FUNCTION "FC_CONVEYORS" : VOID
TITLE =FC DATA EXCHANGE WITH CONVEYOR SYSTEM
{ S7_language := '9(1) Angielski (Stany Zjednoczone)  11.01.2022  09:45:15' }
VERSION : 0.1


VAR_TEMP
  DoorOK : BOOL ;	//ASU COOLING ZONE DOORS OK (CLOSED)
  RET_VAL_IN : INT ;
  RET_VAL_OUT : INT ;
  T_Pos : BOOL ;
  T_Neg : BOOL ;
  FullProd15_Plus1 : REAL ;
  FullProd15_Minus1 : REAL ;
  FullProd20_Plus1 : REAL ;
  FullProd20_Minus1 : REAL ;
END_VAR
BEGIN
NETWORK
TITLE =*********** START ************
//
//******************** INPUT SIGNALS (FROM CONVEYORS) ***************************
//
NETWORK
TITLE =READ DATA FROM CONVEYORS
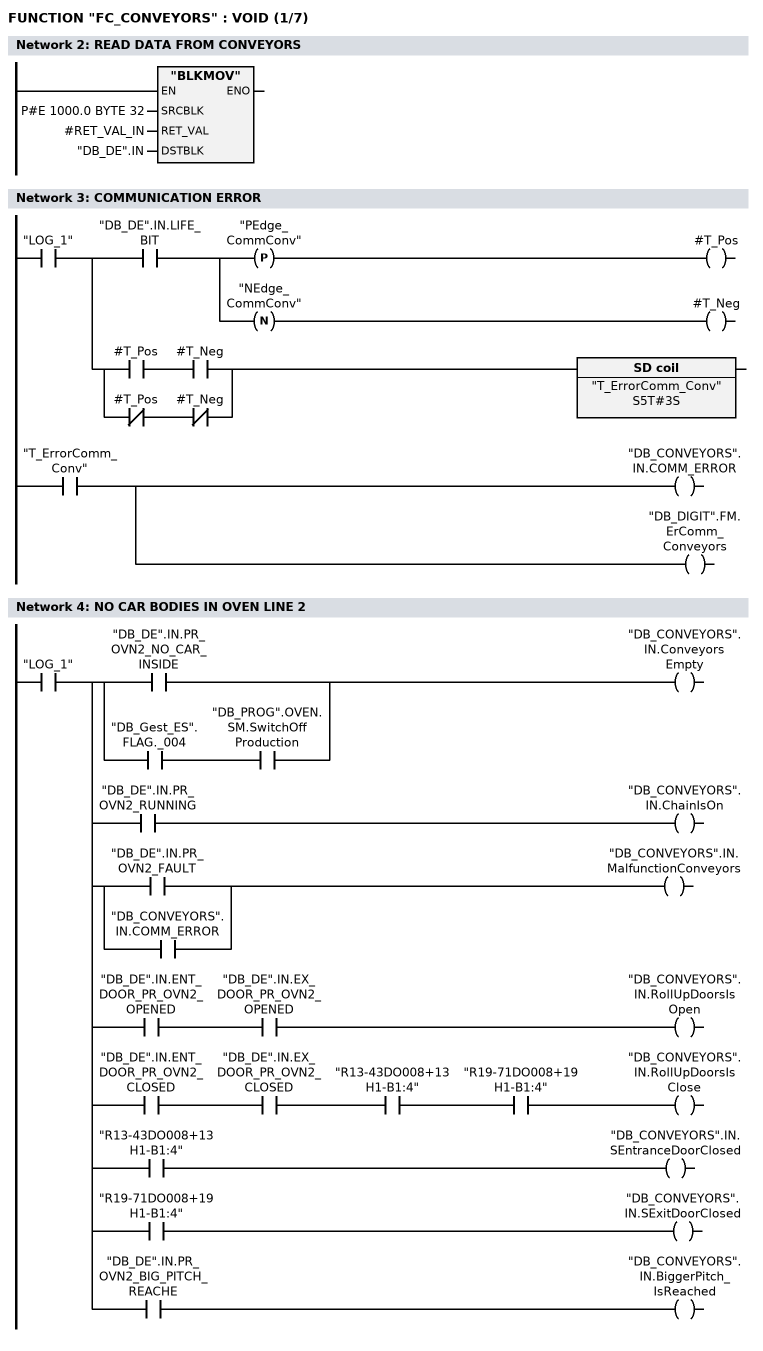
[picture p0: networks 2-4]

      CALL "BLKMOV" (
           SRCBLK                   := P#E 1000.0 BYTE 32,
           RET_VAL                  := #RET_VAL_IN,
           DSTBLK                   := "DB_DE".IN);
      NOP   0;
NETWORK
TITLE =COMMUNICATION ERROR

      U     "LOG_1";
      =     L     24.0;
      U     L     24.0;
      U     "DB_DE".IN.LIFE_BIT;
      =     L     24.1;
      U     L     24.1;
      FP    "PEdge_CommConv";
      =     #T_Pos;
      U     L     24.1;
      FN    "NEdge_CommConv";
      =     #T_Neg;
      U     L     24.0;
      U(    ;
      U     #T_Pos;
      U     #T_Neg;
      O     ;
      UN    #T_Pos;
      UN    #T_Neg;
      )     ;
      L     S5T#3S;
      SE    "T_ErrorComm_Conv";
      NOP   0;
      NOP   0;
      NOP   0;
      U     "T_ErrorComm_Conv";
      =     "DB_CONVEYORS".IN.COMM_ERROR;
      =     "DB_DIGIT".FM.ErComm_Conveyors;
NETWORK
TITLE =NO CAR BODIES IN OVEN LINE 2

      U     "LOG_1";
      =     L     24.0;
      U     L     24.0;
      U(    ;
      O     "DB_DE".IN.PR_OVN2_NO_CAR_INSIDE;
      O     ;
      U     "DB_Gest_ES".FLAG._004;
      U     "DB_PROG".OVEN.SM.SwitchOffProduction;
      )     ;
      =     "DB_CONVEYORS".IN.ConveyorsEmpty;
      U     L     24.0;
      U     "DB_DE".IN.PR_OVN2_RUNNING;
      =     "DB_CONVEYORS".IN.ChainIsOn;
      U     L     24.0;
      U(    ;
      O     "DB_DE".IN.PR_OVN2_FAULT;
      O     "DB_CONVEYORS".IN.COMM_ERROR;
      )     ;
      =     "DB_CONVEYORS".IN.MalfunctionConveyors;
      U     L     24.0;
      U     "DB_DE".IN.ENT_DOOR_PR_OVN2_OPENED;
      U     "DB_DE".IN.EX_DOOR_PR_OVN2_OPENED;
      =     "DB_CONVEYORS".IN.RollUpDoorsIsOpen;
      U     L     24.0;
      U     "DB_DE".IN.ENT_DOOR_PR_OVN2_CLOSED;
      U     "DB_DE".IN.EX_DOOR_PR_OVN2_CLOSED;
      U     "R13-43DO008+13H1-B1:4";
      U     "R19-71DO008+19H1-B1:4";
      =     "DB_CONVEYORS".IN.RollUpDoorsIsClose;
      U     L     24.0;
      U     "R13-43DO008+13H1-B1:4";
      =     "DB_CONVEYORS".IN.SEntranceDoorClosed;
      U     L     24.0;
      U     "R19-71DO008+19H1-B1:4";
      =     "DB_CONVEYORS".IN.SExitDoorClosed;
      U     L     24.0;
      U     "DB_DE".IN.PR_OVN2_BIG_PITCH_REACHE;
      =     "DB_CONVEYORS".IN.BiggerPitch_IsReached;
NETWORK
TITLE =ROLL UP DOOR ENTRANCE IS MOVED FREE
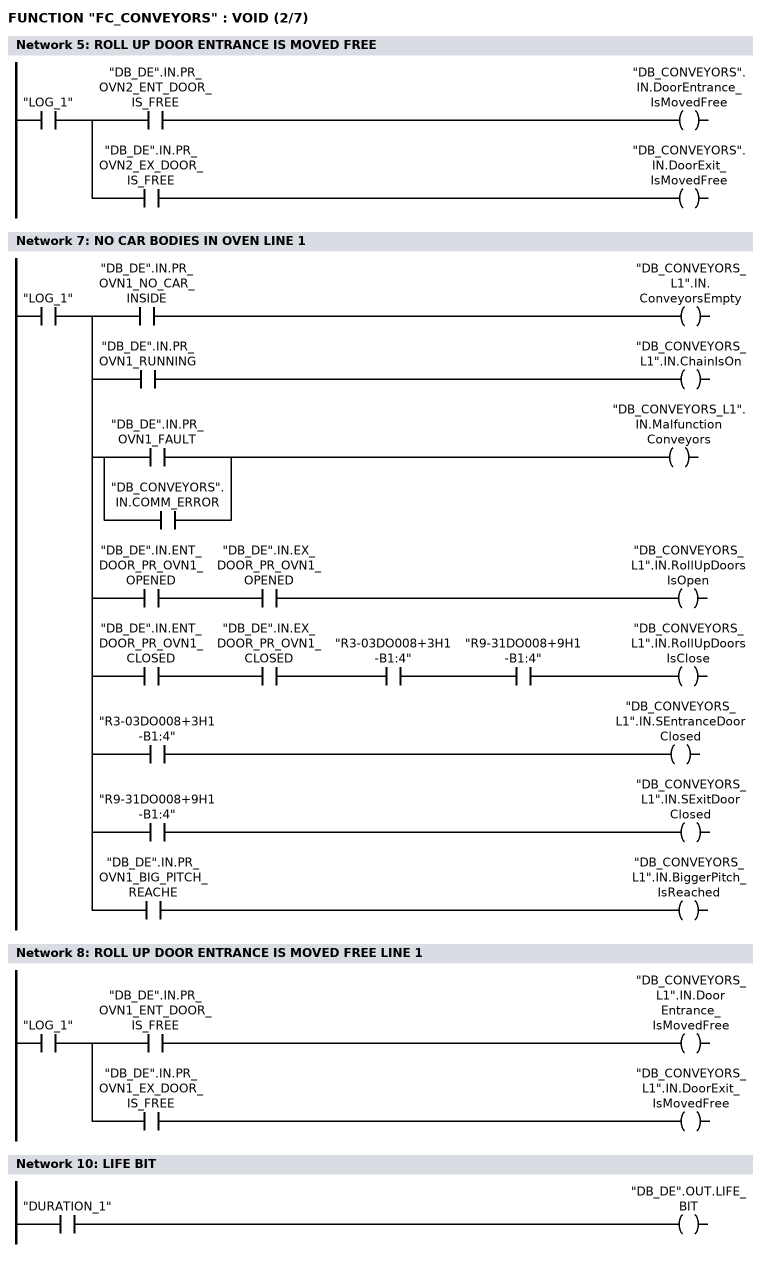
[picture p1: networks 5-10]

      U     "LOG_1";
      =     L     24.0;
      U     L     24.0;
      U     "DB_DE".IN.PR_OVN2_ENT_DOOR_IS_FREE;
      =     "DB_CONVEYORS".IN.DoorEntrance_IsMovedFree;
      U     L     24.0;
      U     "DB_DE".IN.PR_OVN2_EX_DOOR_IS_FREE;
      =     "DB_CONVEYORS".IN.DoorExit_IsMovedFree;
NETWORK
TITLE =LINE 1
//
//****************************** LINE 1 ***********************************
//
NETWORK
TITLE =NO CAR BODIES IN OVEN LINE 1

      U     "LOG_1";
      =     L     24.0;
      U     L     24.0;
      U     "DB_DE".IN.PR_OVN1_NO_CAR_INSIDE;
      =     "DB_CONVEYORS_L1".IN.ConveyorsEmpty;
      U     L     24.0;
      U     "DB_DE".IN.PR_OVN1_RUNNING;
      =     "DB_CONVEYORS_L1".IN.ChainIsOn;
      U     L     24.0;
      U(    ;
      O     "DB_DE".IN.PR_OVN1_FAULT;
      O     "DB_CONVEYORS".IN.COMM_ERROR;
      )     ;
      =     "DB_CONVEYORS_L1".IN.MalfunctionConveyors;
      U     L     24.0;
      U     "DB_DE".IN.ENT_DOOR_PR_OVN1_OPENED;
      U     "DB_DE".IN.EX_DOOR_PR_OVN1_OPENED;
      =     "DB_CONVEYORS_L1".IN.RollUpDoorsIsOpen;
      U     L     24.0;
      U     "DB_DE".IN.ENT_DOOR_PR_OVN1_CLOSED;
      U     "DB_DE".IN.EX_DOOR_PR_OVN1_CLOSED;
      U     "R3-03DO008+3H1-B1:4";
      U     "R9-31DO008+9H1-B1:4";
      =     "DB_CONVEYORS_L1".IN.RollUpDoorsIsClose;
      U     L     24.0;
      U     "R3-03DO008+3H1-B1:4";
      =     "DB_CONVEYORS_L1".IN.SEntranceDoorClosed;
      U     L     24.0;
      U     "R9-31DO008+9H1-B1:4";
      =     "DB_CONVEYORS_L1".IN.SExitDoorClosed;
      U     L     24.0;
      U     "DB_DE".IN.PR_OVN1_BIG_PITCH_REACHE;
      =     "DB_CONVEYORS_L1".IN.BiggerPitch_IsReached;
NETWORK
TITLE =ROLL UP DOOR ENTRANCE IS MOVED FREE LINE 1

      U     "LOG_1";
      =     L     24.0;
      U     L     24.0;
      U     "DB_DE".IN.PR_OVN1_ENT_DOOR_IS_FREE;
      =     "DB_CONVEYORS_L1".IN.DoorEntrance_IsMovedFree;
      U     L     24.0;
      U     "DB_DE".IN.PR_OVN1_EX_DOOR_IS_FREE;
      =     "DB_CONVEYORS_L1".IN.DoorExit_IsMovedFree;
NETWORK
TITLE =******* OUTPUT SIGNALS (TO CONVEYORS) ********
//
//************************** OUTPUT SIGNALS (TO CONVEYORS) **********************
//
NETWORK
TITLE =LIFE BIT

      U     "DURATION_1";
      =     "DB_DE".OUT.LIFE_BIT;
NETWORK
TITLE =SET FULL PRODUCTION OR REDUCED PRODUCTION MODE
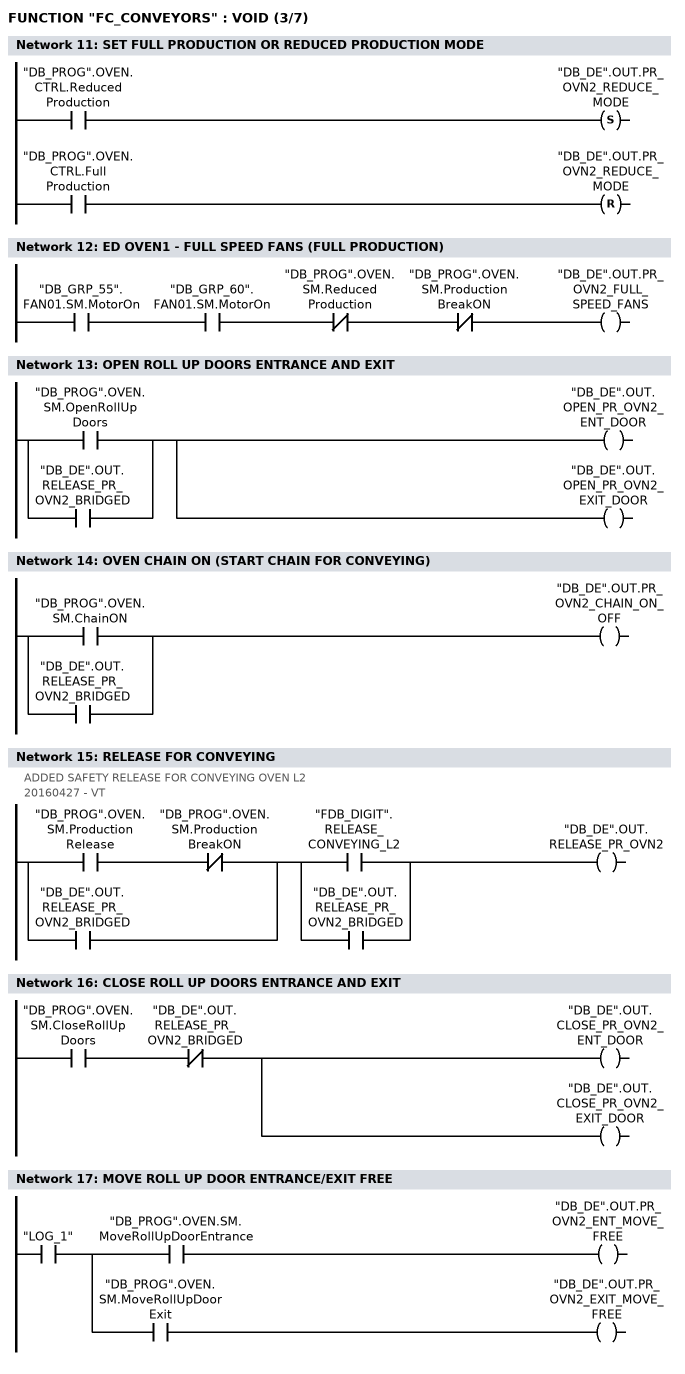
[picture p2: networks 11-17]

      U     "DB_PROG".OVEN.CTRL.ReducedProduction;
      S     "DB_DE".OUT.PR_OVN2_REDUCE_MODE;
      U     "DB_PROG".OVEN.CTRL.FullProduction;
      R     "DB_DE".OUT.PR_OVN2_REDUCE_MODE;
      NOP   0;
NETWORK
TITLE =ED OVEN1 - FULL SPEED FANS (FULL PRODUCTION)

      U     "DB_GRP_55".FAN01.SM.MotorOn;
      U     "DB_GRP_60".FAN01.SM.MotorOn;
      UN    "DB_PROG".OVEN.SM.ReducedProduction;
      UN    "DB_PROG".OVEN.SM.ProductionBreakON;
      =     "DB_DE".OUT.PR_OVN2_FULL_SPEED_FANS;
NETWORK
TITLE =OPEN ROLL UP DOORS ENTRANCE AND EXIT

      O     "DB_PROG".OVEN.SM.OpenRollUpDoors;
      O     "DB_DE".OUT.RELEASE_PR_OVN2_BRIDGED;
      =     "DB_DE".OUT.OPEN_PR_OVN2_ENT_DOOR;
      =     "DB_DE".OUT.OPEN_PR_OVN2_EXIT_DOOR;
NETWORK
TITLE =OVEN CHAIN ON (START CHAIN FOR CONVEYING)

      O     "DB_PROG".OVEN.SM.ChainON;
      O     "DB_DE".OUT.RELEASE_PR_OVN2_BRIDGED;
      =     "DB_DE".OUT.PR_OVN2_CHAIN_ON_OFF;
NETWORK
TITLE =RELEASE FOR CONVEYING
//ADDED SAFETY RELEASE FOR CONVEYING OVEN L2
//
//20160427 - VT
      U(    ;
      U     "DB_PROG".OVEN.SM.ProductionRelease;
      UN    "DB_PROG".OVEN.SM.ProductionBreakON;
      O     "DB_DE".OUT.RELEASE_PR_OVN2_BRIDGED;
      )     ;
      U(    ;
      O     "FDB_DIGIT".RELEASE_CONVEYING_L2;
      O     "DB_DE".OUT.RELEASE_PR_OVN2_BRIDGED;
      )     ;
      =     "DB_DE".OUT.RELEASE_PR_OVN2;
NETWORK
TITLE =CLOSE ROLL UP DOORS ENTRANCE AND EXIT

      U     "DB_PROG".OVEN.SM.CloseRollUpDoors;
      UN    "DB_DE".OUT.RELEASE_PR_OVN2_BRIDGED;
      =     "DB_DE".OUT.CLOSE_PR_OVN2_ENT_DOOR;
      =     "DB_DE".OUT.CLOSE_PR_OVN2_EXIT_DOOR;
NETWORK
TITLE =MOVE ROLL UP DOOR ENTRANCE/EXIT FREE

      U     "LOG_1";
      =     L     24.0;
      U     L     24.0;
      U     "DB_PROG".OVEN.SM.MoveRollUpDoorEntrance;
      =     "DB_DE".OUT.PR_OVN2_ENT_MOVE_FREE;
      U     L     24.0;
      U     "DB_PROG".OVEN.SM.MoveRollUpDoorExit;
      =     "DB_DE".OUT.PR_OVN2_EXIT_MOVE_FREE;
NETWORK
TITLE =LINE 1
//
//*************************** LINE 1 ***************************************
//
NETWORK
TITLE =SET FULL PRODUCTION OR REDUCED PRODUCTION MODE LINE 1
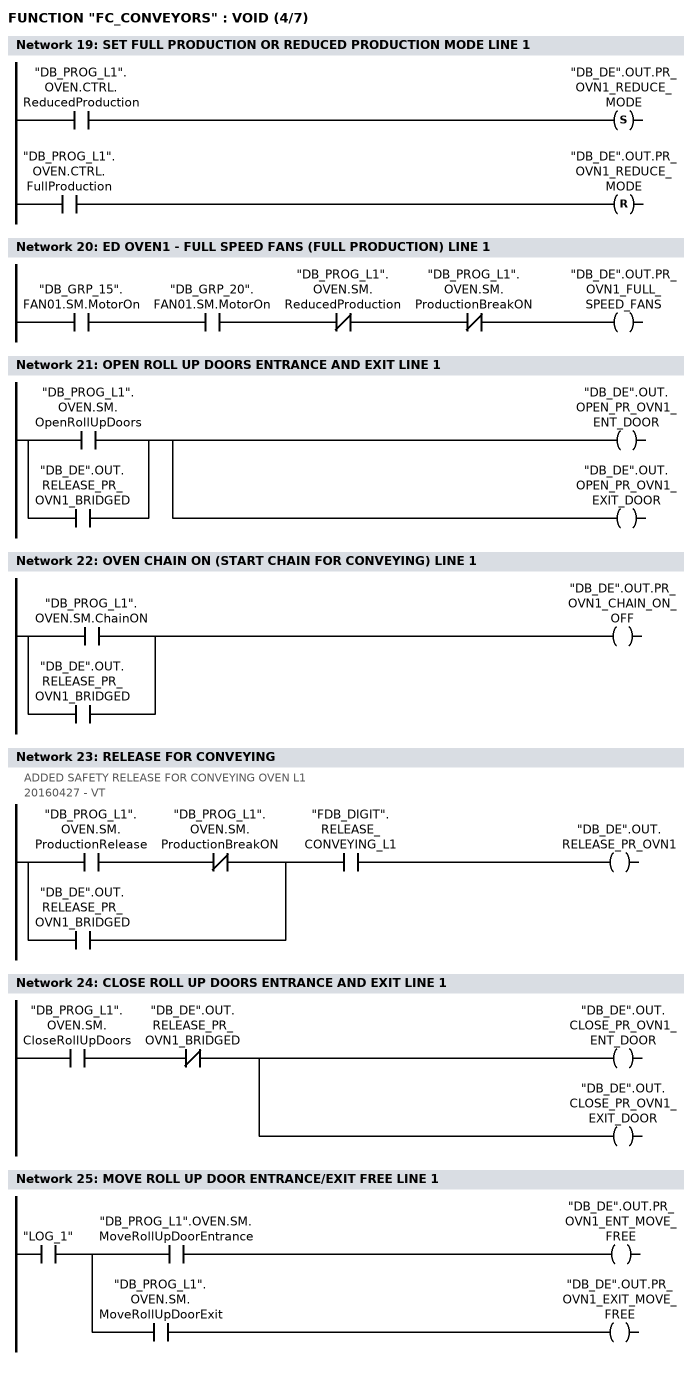
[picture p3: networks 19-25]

      U     "DB_PROG_L1".OVEN.CTRL.ReducedProduction;
      S     "DB_DE".OUT.PR_OVN1_REDUCE_MODE;
      U     "DB_PROG_L1".OVEN.CTRL.FullProduction;
      R     "DB_DE".OUT.PR_OVN1_REDUCE_MODE;
      NOP   0;
NETWORK
TITLE =ED OVEN1 - FULL SPEED FANS (FULL PRODUCTION) LINE 1

      U     "DB_GRP_15".FAN01.SM.MotorOn;
      U     "DB_GRP_20".FAN01.SM.MotorOn;
      UN    "DB_PROG_L1".OVEN.SM.ReducedProduction;
      UN    "DB_PROG_L1".OVEN.SM.ProductionBreakON;
      =     "DB_DE".OUT.PR_OVN1_FULL_SPEED_FANS;
NETWORK
TITLE =OPEN ROLL UP DOORS ENTRANCE AND EXIT LINE 1

      O     "DB_PROG_L1".OVEN.SM.OpenRollUpDoors;
      O     "DB_DE".OUT.RELEASE_PR_OVN1_BRIDGED;
      =     "DB_DE".OUT.OPEN_PR_OVN1_ENT_DOOR;
      =     "DB_DE".OUT.OPEN_PR_OVN1_EXIT_DOOR;
NETWORK
TITLE =OVEN CHAIN ON (START CHAIN FOR CONVEYING) LINE 1

      O     "DB_PROG_L1".OVEN.SM.ChainON;
      O     "DB_DE".OUT.RELEASE_PR_OVN1_BRIDGED;
      =     "DB_DE".OUT.PR_OVN1_CHAIN_ON_OFF;
NETWORK
TITLE =RELEASE FOR CONVEYING
//ADDED SAFETY RELEASE FOR CONVEYING OVEN L1
//
//20160427 - VT
      U(    ;
      U     "DB_PROG_L1".OVEN.SM.ProductionRelease;
      UN    "DB_PROG_L1".OVEN.SM.ProductionBreakON;
      O     "DB_DE".OUT.RELEASE_PR_OVN1_BRIDGED;
      )     ;
      U     "FDB_DIGIT".RELEASE_CONVEYING_L1;
      =     "DB_DE".OUT.RELEASE_PR_OVN1;
NETWORK
TITLE =CLOSE ROLL UP DOORS ENTRANCE AND EXIT LINE 1

      U     "DB_PROG_L1".OVEN.SM.CloseRollUpDoors;
      UN    "DB_DE".OUT.RELEASE_PR_OVN1_BRIDGED;
      =     "DB_DE".OUT.CLOSE_PR_OVN1_ENT_DOOR;
      =     "DB_DE".OUT.CLOSE_PR_OVN1_EXIT_DOOR;
NETWORK
TITLE =MOVE ROLL UP DOOR ENTRANCE/EXIT FREE LINE 1

      U     "LOG_1";
      =     L     24.0;
      U     L     24.0;
      U     "DB_PROG_L1".OVEN.SM.MoveRollUpDoorEntrance;
      =     "DB_DE".OUT.PR_OVN1_ENT_MOVE_FREE;
      U     L     24.0;
      U     "DB_PROG_L1".OVEN.SM.MoveRollUpDoorExit;
      =     "DB_DE".OUT.PR_OVN1_EXIT_MOVE_FREE;
NETWORK
TITLE =*********** NPL - COMMUNICATION **************
//
//*******************************************************************************
//
//                     EXCHANGE SIGNALS WITH FIAT FACTORY
//                           NPL - COMMUNICATION
//
//******************************************************************************
NETWORK
TITLE =NPL SIGNALS
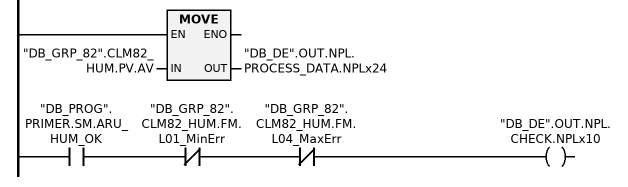
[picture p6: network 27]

//NPL PROCESS DATA
//NPL OVEN LINE1
      L     "DB_GRP_00".RIT12.PV.AV;
      T     "DB_DE".OUT.NPL.PROCESS_DATA.NPLx01;
      UN    "DB_GRP_00".RIT12.FM.L01_MinErr;
      UN    "DB_GRP_00".RIT12.FM.L04_MaxErr;
      =     "DB_DE".OUT.NPL.CHECK.NPLx01;

      L     "DB_GRP_00".RIT13.PV.AV;
      T     "DB_DE".OUT.NPL.PROCESS_DATA.NPLx02;
      UN    "DB_GRP_00".RIT13.FM.L01_MinErr;
      UN    "DB_GRP_00".RIT13.FM.L04_MaxErr;
      =     "DB_DE".OUT.NPL.CHECK.NPLx02;

      L     "DB_GRP_00".RIT15.PV.AV;
      T     "DB_DE".OUT.NPL.PROCESS_DATA.NPLx03;
      U     "TempOK_GRP_03";
      UN    "DB_GRP_00".RIT15.FM.L01_MinErr;
      UN    "DB_GRP_00".RIT15.FM.L04_MaxErr;
      =     "DB_DE".OUT.NPL.CHECK.NPLx03;

      L     "DB_GRP_00".RIT16.PV.AV;
      T     "DB_DE".OUT.NPL.PROCESS_DATA.NPLx04;
      U     "TempOK_GRP_04";
      UN    "DB_GRP_00".RIT16.FM.L01_MinErr;
      UN    "DB_GRP_00".RIT16.FM.L04_MaxErr;
      =     "DB_DE".OUT.NPL.CHECK.NPLx04;

      L     "DB_GRP_00".RIT17.PV.AV;
      T     "DB_DE".OUT.NPL.PROCESS_DATA.NPLx05;
      U     "TempOK_GRP_11";
      UN    "DB_GRP_00".RIT17.FM.L01_MinErr;
      UN    "DB_GRP_00".RIT17.FM.L04_MaxErr;
      =     "DB_DE".OUT.NPL.CHECK.NPLx05;

      L     "DB_GRP_00".RIT18.PV.AV;
      T     "DB_DE".OUT.NPL.PROCESS_DATA.NPLx06;
      U     "TempOK_GRP_12";
      UN    "DB_GRP_00".RIT15.FM.L01_MinErr;
      UN    "DB_GRP_00".RIT15.FM.L04_MaxErr;
      =     "DB_DE".OUT.NPL.CHECK.NPLx06;

//NPL OVEN LINE2
      L     "DB_GRP_40".RIT12.PV.AV;
      T     "DB_DE".OUT.NPL.PROCESS_DATA.NPLx11;
      UN    "DB_GRP_40".RIT12.FM.L01_MinErr;
      UN    "DB_GRP_40".RIT12.FM.L04_MaxErr;
      =     "DB_DE".OUT.NPL.CHECK.NPLx11;

      L     "DB_GRP_40".RIT13.PV.AV;
      T     "DB_DE".OUT.NPL.PROCESS_DATA.NPLx12;
      UN    "DB_GRP_40".RIT13.FM.L01_MinErr;
      UN    "DB_GRP_40".RIT13.FM.L04_MaxErr;
      =     "DB_DE".OUT.NPL.CHECK.NPLx12;

      L     "DB_GRP_40".RIT15.PV.AV;
      T     "DB_DE".OUT.NPL.PROCESS_DATA.NPLx13;
      U     "TempOK_GRP_43";
      UN    "DB_GRP_40".RIT15.FM.L01_MinErr;
      UN    "DB_GRP_40".RIT15.FM.L04_MaxErr;
      =     "DB_DE".OUT.NPL.CHECK.NPLx13;

      L     "DB_GRP_40".RIT16.PV.AV;
      T     "DB_DE".OUT.NPL.PROCESS_DATA.NPLx14;
      U     "TempOK_GRP_44";
      UN    "DB_GRP_40".RIT16.FM.L01_MinErr;
      UN    "DB_GRP_40".RIT16.FM.L04_MaxErr;
      =     "DB_DE".OUT.NPL.CHECK.NPLx14;

      L     "DB_GRP_40".RIT17.PV.AV;
      T     "DB_DE".OUT.NPL.PROCESS_DATA.NPLx15;
      U     "TempOK_GRP_51";
      UN    "DB_GRP_40".RIT17.FM.L01_MinErr;
      UN    "DB_GRP_40".RIT17.FM.L04_MaxErr;
      =     "DB_DE".OUT.NPL.CHECK.NPLx15;

      L     "DB_GRP_40".RIT18.PV.AV;
      T     "DB_DE".OUT.NPL.PROCESS_DATA.NPLx16;
      U     "TempOK_GRP_52";
      UN    "DB_GRP_40".RIT18.FM.L01_MinErr;
      UN    "DB_GRP_40".RIT18.FM.L04_MaxErr;
      =     "DB_DE".OUT.NPL.CHECK.NPLx16;

//NPL PRIMER BOOTH
      L     "DB_GRP_81".CLT81.PV.AV;
      T     "DB_DE".OUT.NPL.PROCESS_DATA.NPLx21;
      U     "DB_PROG".PRIMER.SM.ASU_TEMP_OK;
      UN    "DB_GRP_81".CLT81.FM.L01_MinErr;
      UN    "DB_GRP_81".CLT81.FM.L04_MaxErr;
      =     "DB_DE".OUT.NPL.CHECK.NPLx07;

      L     "DB_GRP_81".CLM82_HUM.PV.AV;
      T     "DB_DE".OUT.NPL.PROCESS_DATA.NPLx22;
      U     "DB_PROG".PRIMER.SM.ASU_HUM_OK;
      UN    "DB_GRP_81".CLM82_HUM.FM.L01_MinErr;
      UN    "DB_GRP_81".CLM82_HUM.FM.L04_MaxErr;
      =     "DB_DE".OUT.NPL.CHECK.NPLx08;

      L     "DB_GRP_82".CLT81.PV.AV;
      T     "DB_DE".OUT.NPL.PROCESS_DATA.NPLx23;
      U     "DB_PROG".PRIMER.SM.ARU_TEMP_OK;
      UN    "DB_GRP_82".CLT81.FM.L01_MinErr;
      UN    "DB_GRP_82".CLT81.FM.L04_MaxErr;
      =     "DB_DE".OUT.NPL.CHECK.NPLx09;

      L     "DB_GRP_82".CLM82_HUM.PV.AV;
      T     "DB_DE".OUT.NPL.PROCESS_DATA.NPLx24;
      U     "DB_PROG".PRIMER.SM.ARU_HUM_OK;
      UN    "DB_GRP_82".CLM82_HUM.FM.L01_MinErr;
      UN    "DB_GRP_82".CLM82_HUM.FM.L04_MaxErr;
      =     "DB_DE".OUT.NPL.CHECK.NPLx10;

NETWORK
TITLE =*********** END ************
//
//******************** OUTPUT SIGNALS (TO CONVEYORS) ***************************
//
NETWORK
TITLE =

NETWORK
TITLE =INTERLOCKS - PLC CONVEYORS --> FLASH-OFF SYSTEM
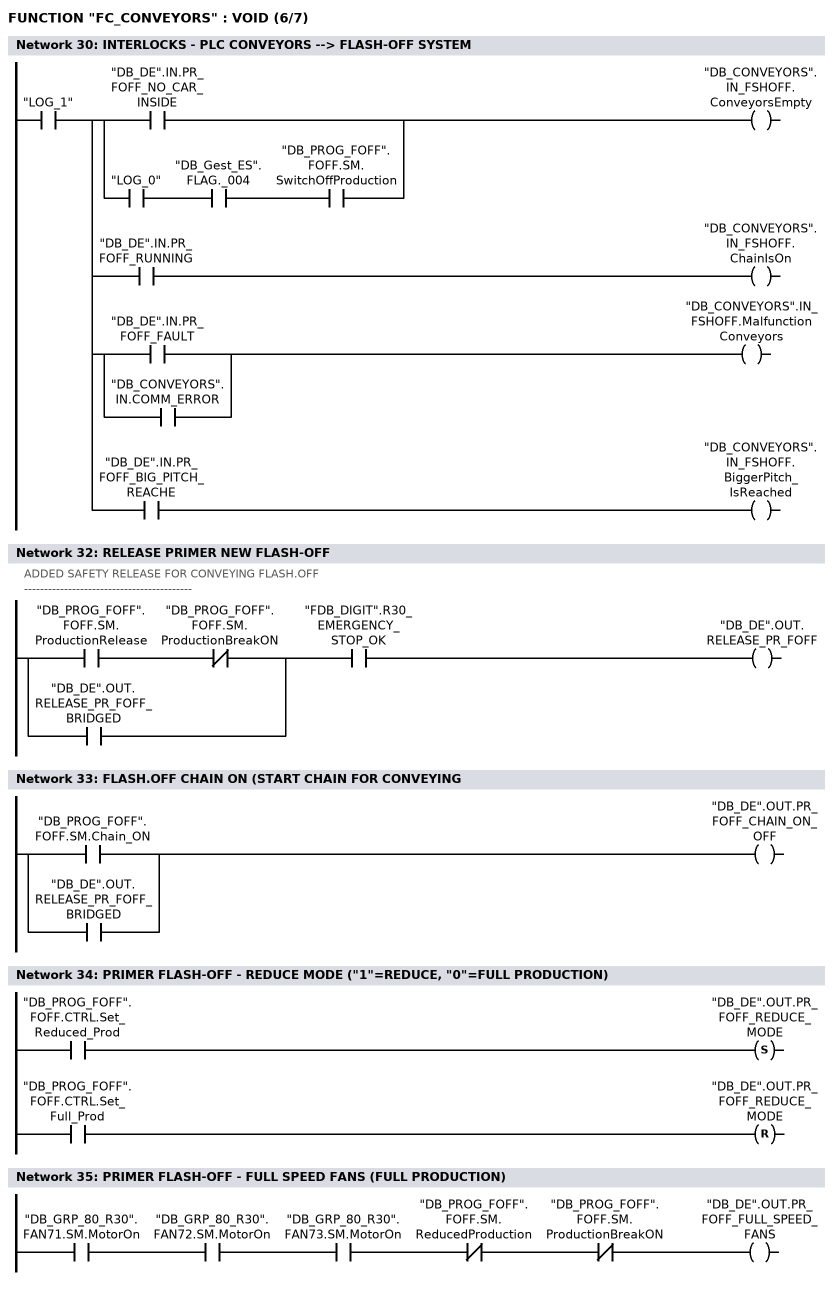
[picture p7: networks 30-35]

      U     "LOG_1";
      =     L     24.0;
      U     L     24.0;
      U(    ;
      O     "DB_DE".IN.PR_FOFF_NO_CAR_INSIDE;
      O     ;
      U     "LOG_0";
      U     "DB_Gest_ES".FLAG._004;
      U     "DB_PROG_FOFF".FOFF.SM.SwitchOffProduction;
      )     ;
      =     "DB_CONVEYORS".IN_FSHOFF.ConveyorsEmpty;
      U     L     24.0;
      U     "DB_DE".IN.PR_FOFF_RUNNING;
      =     "DB_CONVEYORS".IN_FSHOFF.ChainIsOn;
      U     L     24.0;
      U(    ;
      O     "DB_DE".IN.PR_FOFF_FAULT;
      O     "DB_CONVEYORS".IN.COMM_ERROR;
      )     ;
      =     "DB_CONVEYORS".IN_FSHOFF.MalfunctionConveyors;
      U     L     24.0;
      U     "DB_DE".IN.PR_FOFF_BIG_PITCH_REACHE;
      =     "DB_CONVEYORS".IN_FSHOFF.BiggerPitch_IsReached;
NETWORK
TITLE =INTERLOCKS - FLASH-OFF SYSTEM --> PLC CONVEYORS

NETWORK
TITLE =RELEASE PRIMER NEW FLASH-OFF
//ADDED SAFETY RELEASE FOR CONVEYING FLASH.OFF
//------------------------------------------
      U(    ;
      U     "DB_PROG_FOFF".FOFF.SM.ProductionRelease;
      UN    "DB_PROG_FOFF".FOFF.SM.ProductionBreakON;
      O     "DB_DE".OUT.RELEASE_PR_FOFF_BRIDGED;
      )     ;
      U     "FDB_DIGIT".R30_EMERGENCY_STOP_OK;
      =     "DB_DE".OUT.RELEASE_PR_FOFF;
NETWORK
TITLE =FLASH.OFF CHAIN ON (START CHAIN FOR CONVEYING

      O     "DB_PROG_FOFF".FOFF.SM.Chain_ON;
      O     "DB_DE".OUT.RELEASE_PR_FOFF_BRIDGED;
      =     "DB_DE".OUT.PR_FOFF_CHAIN_ON_OFF;
NETWORK
TITLE =PRIMER FLASH-OFF - REDUCE MODE ("1"=REDUCE, "0"=FULL PRODUCTION)

      U     "DB_PROG_FOFF".FOFF.CTRL.Set_Reduced_Prod;
      S     "DB_DE".OUT.PR_FOFF_REDUCE_MODE;
      U     "DB_PROG_FOFF".FOFF.CTRL.Set_Full_Prod;
      R     "DB_DE".OUT.PR_FOFF_REDUCE_MODE;
      NOP   0;
NETWORK
TITLE =PRIMER FLASH-OFF - FULL SPEED FANS (FULL PRODUCTION)

      U     "DB_GRP_80_R30".FAN71.SM.MotorOn;
      U     "DB_GRP_80_R30".FAN72.SM.MotorOn;
      U     "DB_GRP_80_R30".FAN73.SM.MotorOn;
      UN    "DB_PROG_FOFF".FOFF.SM.ReducedProduction;
      UN    "DB_PROG_FOFF".FOFF.SM.ProductionBreakON;
      =     "DB_DE".OUT.PR_FOFF_FULL_SPEED_FANS;
NETWORK
TITLE =

NETWORK
TITLE =
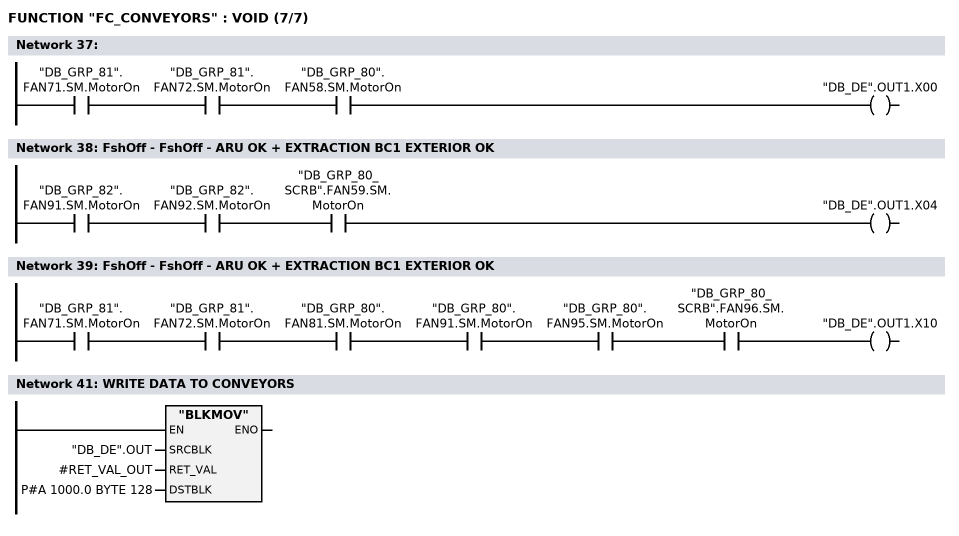
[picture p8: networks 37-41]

      U     "DB_GRP_81".FAN71.SM.MotorOn;
      U     "DB_GRP_81".FAN72.SM.MotorOn;
      U     "DB_GRP_80".FAN58.SM.MotorOn;
      =     "DB_DE".OUT1.X00;
NETWORK
TITLE =FshOff - FshOff - ARU OK + EXTRACTION BC1 EXTERIOR OK

      U     "DB_GRP_82".FAN91.SM.MotorOn;
      U     "DB_GRP_82".FAN92.SM.MotorOn;
      U     "DB_GRP_80_SCRB".FAN59.SM.MotorOn;
      =     "DB_DE".OUT1.X04;
NETWORK
TITLE =FshOff - FshOff - ARU OK + EXTRACTION BC1 EXTERIOR OK

      U     "DB_GRP_81".FAN71.SM.MotorOn;
      U     "DB_GRP_81".FAN72.SM.MotorOn;
      U     "DB_GRP_80".FAN81.SM.MotorOn;
      U     "DB_GRP_80".FAN91.SM.MotorOn;
      U     "DB_GRP_80".FAN95.SM.MotorOn;
      U     "DB_GRP_80_SCRB".FAN96.SM.MotorOn;
      =     "DB_DE".OUT1.X10;
NETWORK
TITLE =

NETWORK
TITLE =WRITE DATA TO CONVEYORS

      CALL "BLKMOV" (
           SRCBLK                   := "DB_DE".OUT,
           RET_VAL                  := #RET_VAL_OUT,
           DSTBLK                   := P#A 1000.0 BYTE 128);
      NOP   0;
NETWORK
TITLE =END

END_FUNCTION

